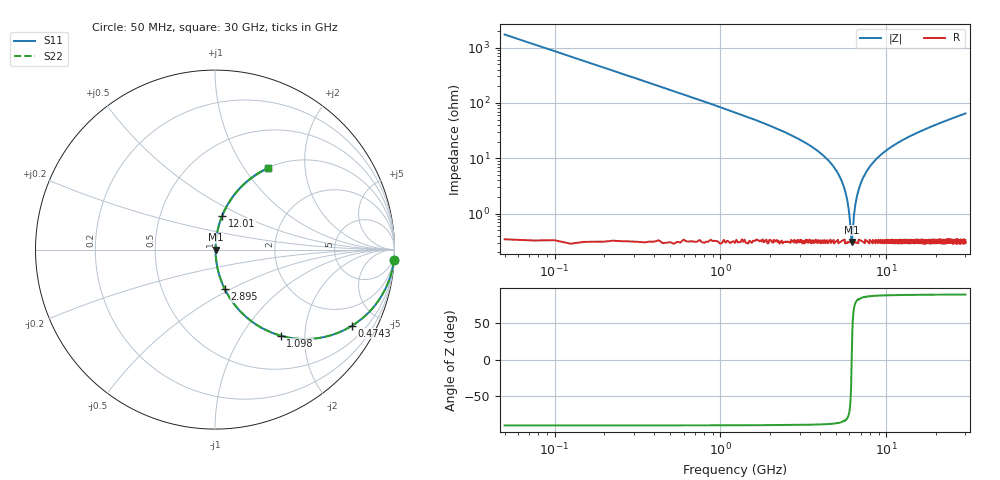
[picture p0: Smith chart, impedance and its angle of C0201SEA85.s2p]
!	AVX Thin Film Operation 	Date: April 2014
!	Description: Accu-P® Series, Thin Film  SMD RF Capacitor
!	Part Number: 02013JA85PBSTR
# MHZ S MA R 50
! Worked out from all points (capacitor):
!   1201 points, 50 MHz to 30 GHz, reference 50 ohm
!   read as one part in series: C = 1.85 pF near 199.8 MHz
!   lowest |Z| = 309 mohm at 6.19 GHz (marker M1)
!   series resonance near 6.189 GHz, so ESL is about 360 pH
!   S11 on the Smith chart (normalised r, x): 50 MHz: 1, -34; 474.3 MHz: 1.01, -3.61; 1.098 GHz: 1.01, -1.52; 2.895 GHz: 1.01, -0.46; 12.01 GHz: 1.01, +0.40; 30 GHz: 1.01, +1.29
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50  0.998 -3.3  0.058 86.7  0.058 86.7  0.998 -3.3
274.625  0.952 -17.7  0.305 72.2  0.305 72.2  0.952 -17.7
474.292  0.874 -29.0  0.485 60.9  0.485 60.9  0.874 -29.0
1098.25  0.603 -52.7  0.795 37.1  0.795 37.1  0.603 -52.7
1797.083  0.4 -66.0  0.913 23.6  0.913 23.6  0.4 -66.0
2895.25  0.225 -76.2  0.971 13.0  0.971 13.0  0.225 -76.2
5041.667  0.057 -83.6  0.995 3.3  0.995 3.3  0.057 -83.6
5690.583  0.023 -81.0  0.997 1.3  0.997 1.3  0.023 -81.0
5890.25  0.014 -76.3  0.997 0.8  0.997 0.8  0.014 -76.3
6089.917  0.005455 -54.5  0.997 0.3  0.997 0.3  0.005455 -54.5
6189.75  0.003151 1.0  0.997 -0.0  0.997 -0.0  0.003151 1.0
6289.583  0.005483 54.7  0.997 -0.3  0.997 -0.3  0.005483 54.7
6464.292  0.012 74.7  0.997 -0.7  0.997 -0.7  0.012 74.7
6639  0.02 79.7  0.997 -1.1  0.997 -1.1  0.02 79.7
7213.042  0.043 83.3  0.996 -2.4  0.996 -2.4  0.043 83.3
8361.125  0.084 83.0  0.993 -4.8  0.993 -4.8  0.084 83.0
10058.29  0.139 80.7  0.987 -8.0  0.987 -8.0  0.139 80.7
12005.04  0.194 77.9  0.978 -11.2  0.978 -11.2  0.194 77.9
15025  0.269 73.7  0.96 -15.6  0.96 -15.6  0.269 73.7
20016.67  0.376 67.5  0.924 -22.1  0.924 -22.1  0.376 67.5
25033.29  0.466 61.9  0.882 -27.8  0.882 -27.8  0.466 61.9
30000  0.541 57.0  0.838 -32.7  0.838 -32.7  0.541 57.0
